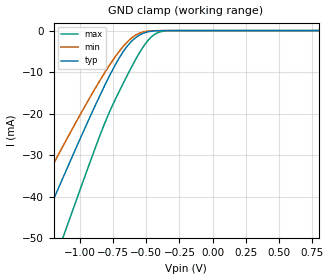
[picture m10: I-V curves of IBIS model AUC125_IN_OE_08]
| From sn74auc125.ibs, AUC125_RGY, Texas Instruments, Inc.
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[Model]   AUC125_IN_OE_08
Model_type  Input
Vinl=0.28
Vinh=0.52
| variable   typ   min   max
C_comp   2.59pF   2.06pF   3.05pF
[Temperature Range]   40   100   -40
| Ambient temperature   25   85   -40
[Voltage range]   0.8   0.8   0.8
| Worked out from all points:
|   GND clamp passes 1 mA (typ) near -0.55 V on its own axis
[GND Clamp]
| AUC125_IN_OE_08
|   Voltage   I(typ)   I(min)   I(max)
-3.6V     -222.6mA   -186.3mA   -267.8mA
-1.5V     -63.1mA    -50.47mA   -83.04mA
-1.455V   -59.72mA   -47.68mA   -79.03mA
-1.325V   -49.98mA   -39.67mA   -67.42mA
-1.28V    -46.63mA   -36.93mA   -63.4mA
-1.12V    -34.83mA   -27.33mA   -49.09mA
-825mV    -13.99mA   -10.73mA   -23.23mA
-695mV    -6.117mA   -4.635mA   -14.06mA
-580mV    -1.725mA   -1.097mA   -6.949mA
-450mV    -123.7uA   -58.74uA   -1.212mA
-315mV    -2.431uA   -1.521uA   -21.15uA
800mV     100.9pA    184.3pA    81.62pA
